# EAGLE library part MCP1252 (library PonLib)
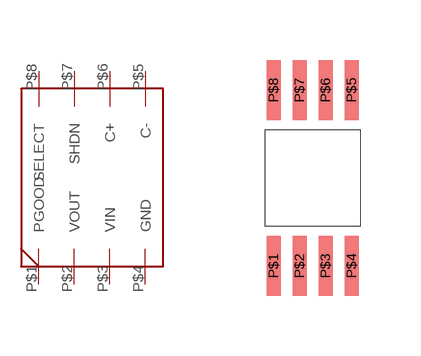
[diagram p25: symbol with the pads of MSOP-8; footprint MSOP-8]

Designator prefix -

## MCP1252  [MSOP-8]
P$1  PGOOD
P$2  VOUT
P$3  VIN
P$4  GND
P$5  C-
P$6  C+
P$7  SHDN
P$8  SELECT

## Footprint MSOP-8 (pad centres in mm)
smd 0.35 x 1.5: P$1 -0.975,-2.2; P$2 -0.325,-2.2; P$3 0.325,-2.2; P$4 0.975,-2.2; P$5 0.975,2.2; P$6 0.325,2.2; P$7 -0.325,2.2; P$8 -0.975,2.2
